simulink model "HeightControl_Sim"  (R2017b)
settings: Solver=ode4  StartTime=0.0  StopTime=2  FixedStep=0.001  RelTol=1e-3
InitFcn:
  | Init_control;
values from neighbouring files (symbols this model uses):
  DEG2RAD = 0.0174533    [Init_control.m]
  Kd_PITCH_AngleRate = 0.001    [Init_control.m]
  Kd_ROLL_AngleRate = 0.001    [Init_control.m]
  Kd_YAW_AngleRate = 0.00    (= 0)    [Init_control.m]
  Ki_PITCH_AngleRate = 0.02    [Init_control.m]
  Ki_ROLL_AngleRate = 0.02    [Init_control.m]
  Ki_YAW_AngleRate = 0.001    [Init_control.m]
  Kp_PITCH_ANGLE = 6.5    [Init_control.m]
  Kp_PITCH_AngleRate = 0.1    [Init_control.m]
  Kp_ROLL_ANGLE = 6.5    [Init_control.m]
  Kp_ROLL_AngleRate = 0.1    [Init_control.m]
  Kp_YAW_AngleRate = 0.3    [Init_control.m]
  Kpxp = 1.0    (= 1)    [Init_control.m]
  Kpyp = 1.0    (= 1)    [Init_control.m]
  Kpzp = 4.0    (= 4)    [Init_control.m]
  Kvxd = 0.01    [Init_control.m]
  Kvxi = 0.4    [Init_control.m]
  Kvxp = 2.5    [Init_control.m]
  Kvyd = 0.01    [Init_control.m]
  Kvyi = 0.4    [Init_control.m]
  Kvyp = 2.5    [Init_control.m]
  Kvzd = 0.005    [Init_control.m]
  Kvzi = 0.01    [Init_control.m]
  Kvzp = 0.45    [Init_control.m]
  MAX_CONTROL_ANGLE_PITCH = 35    [Init_control.m]
  MAX_CONTROL_ANGLE_RATE_PITCH = 220    [Init_control.m]
  MAX_CONTROL_ANGLE_RATE_ROLL = 220    [Init_control.m]
  MAX_CONTROL_ANGLE_RATE_Y = 200    [Init_control.m]
  MAX_CONTROL_ANGLE_ROLL = 35    [Init_control.m]
  MAX_CONTROL_VELOCITY_XY = 5    [Init_control.m]
  MAX_CONTROL_VELOCITY_Z = 3    [Init_control.m]
  ModelInit_AngEuler = [0, 0, 0]    [Init_control.m]    (also in Init.m)
  ModelInit_PosE = [0, 0, -100]    [Init_control.m]    (also in Init.m = [0, 0, 0])
  ModelInit_Rads = 0    [Init_control.m]    (also in Init.m)
  ModelInit_RateB = [0, 0, 0]    [Init_control.m]    (also in Init.m)
  ModelInit_VelB = [0, 0, 0]    [Init_control.m]    (also in Init.m)
  ModelParam_envGravityAcc = 9.8    [Init.m]
  ModelParam_motorCr = 1148    [Init.m]
  ModelParam_motorJm = 0.0001287    [Init.m]
  ModelParam_motorT = 0.02    [Init.m]
  ModelParam_motorWb = -141.4    [Init.m]
  ModelParam_rotorCm = 1.779e-07    [Init.m]
  ModelParam_rotorCt = 1.105e-05    [Init.m]
  ModelParam_uavCCm = [0.0035 0.0039 0.0034]    [Init.m]
  ModelParam_uavCd = 0.055    [Init.m]
  ModelParam_uavJ = [ModelParam_uavJxx, 0, 0;     0, ModelParam_uavJyy, 0;     0, 0, ModelParam_uavJzz]    [Init.m]
  ModelParam_uavMass = 1.4    [Init.m]
  ModelParam_uavR = 0.225    [Init.m]
  Saturation_I_ah = 3.43    [Init_control.m]
  Saturation_I_az = 5    [Init_control.m]
  Saturation_I_RP_Max = 0.3    [Init_control.m]
  Saturation_I_RP_Min = -0.3    [Init_control.m]
  Saturation_I_Y_Max = 0.2    [Init_control.m]
  Saturation_I_Y_Min = -0.2    [Init_control.m]
  THR_HOVER = 0.609    [Init_control.m]
undefined symbols (not defined in the file or in its folder): Column, D, DiscIntNeverNeededParam, earthRadius, Receive, Send, vector
libraries: simulink x8, aerolibfltsims x3, sharedutil x2, aerolibanimutils x1
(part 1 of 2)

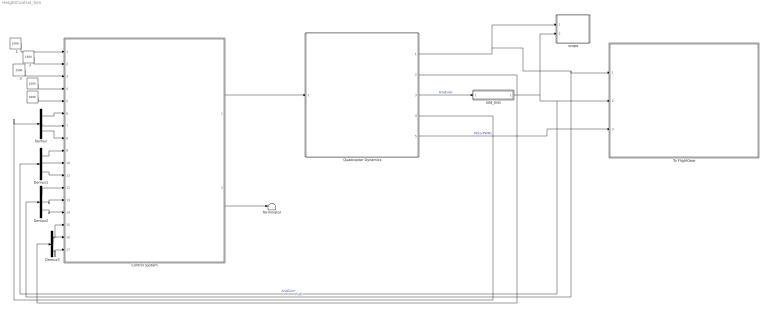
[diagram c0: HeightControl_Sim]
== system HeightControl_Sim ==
  " " : Constant  Value=1000  OutDataTypeStr=uint16
  "          " : Constant  Value=1500  OutDataTypeStr=uint16
  "   1" : Constant  Value=1500  OutDataTypeStr=uint16
  "   2" : Constant  Value=1500  OutDataTypeStr=uint16
  "   3" : Constant  Value=1500  OutDataTypeStr=uint16
  Control System : Subsystem
  Demux{,1..3} (4 alike) : Demux  Outputs=3
  Quadcopter Dynamics : Subsystem
  Terminator : Terminator
  To FlightGear : Subsystem
  add_bias : Subsystem
  scope : Subsystem
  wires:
  Quadcopter Dynamics/1(PosE) -> scope/1(Pos), To FlightGear/1(PosE), Demux2/1  "PosE"
  Quadcopter Dynamics/5(MotorRPMS) -> To FlightGear/3(MotorPWMs)  "MotorPWMs"
  Control System/2(LED) -> Terminator/1
  add_bias/1("eulerAngle ") -> scope/2(EulerAngle), To FlightGear/2(AngEuler), Demux1/1  "AngEuler"
  "          "/1 -> Control System/4(ch4)
  Quadcopter Dynamics/4(AngRateB) -> Demux/1
  " "/1 -> Control System/5(ch5)
  Demux/1 -> Control System/6(p)
  Demux/2 -> Control System/7(q)
  Demux/3 -> Control System/8(r)
  Demux2/1 -> Control System/12(x)
  Demux2/2 -> Control System/13(y)
  Demux2/3 -> Control System/14(z)
  Demux3/1 -> Control System/15(vx)
  Demux3/2 -> Control System/16(vy)
  Demux3/3 -> Control System/17(vz)
  "   1"/1 -> Control System/1(ch1)
  Quadcopter Dynamics/2(VelE) -> Demux3/1
  "   2"/1 -> Control System/2(ch2)
  Quadcopter Dynamics/3(AngEuler) -> add_bias/1(eulerAngle)  "AngEuler"
  Demux1/2 -> Control System/10(pitch)
  Demux1/1 -> Control System/9(roll)
  Demux1/3 -> Control System/11(yaw)
  "   3"/1 -> Control System/3(ch3)
  Control System/1(PWM) -> Quadcopter Dynamics/1(inPWMs)

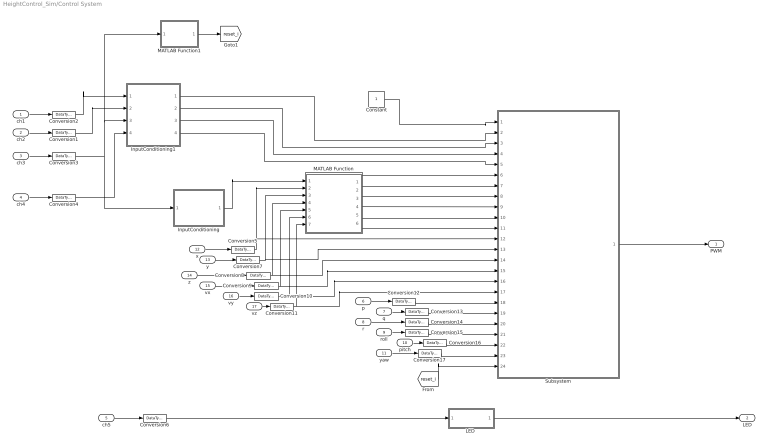
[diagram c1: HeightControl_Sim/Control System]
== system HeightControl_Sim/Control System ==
  ch1 : Inport  OutDataTypeStr=uint16  PortDimensions=1
  ch2 : Inport  Port=2  OutDataTypeStr=uint16  PortDimensions=1
  ch3 : Inport  Port=3  OutDataTypeStr=uint16  PortDimensions=1
  ch4 : Inport  Port=4  OutDataTypeStr=uint16  PortDimensions=1
  ch5 : Inport  Port=5  OutDataTypeStr=uint16  PortDimensions=1  Interpolate=off
  p : Inport  Port=6  PortDimensions=1
  q : Inport  Port=7  PortDimensions=1
  r : Inport  Port=8  PortDimensions=1
  roll : Inport  Port=9  PortDimensions=1
  pitch : Inport  Port=10  PortDimensions=1
  yaw : Inport  Port=11  PortDimensions=1
  x : Inport  Port=12
  y : Inport  Port=13
  z : Inport  Port=14
  vx : Inport  Port=15
  vy : Inport  Port=16
  vz : Inport  Port=17
  Constant : Constant
  Conversion{1..17} (17 alike) : DataTypeConversion  OutDataTypeStr=double
  InputConditioning : Subsystem
  InputConditioning1 : Subsystem
  "LED " : Subsystem
  MATLAB Function : MATLAB Function
  MATLAB Function1 : MATLAB Function  TreatAsAtomicUnit=on
  Subsystem : Subsystem
  PWM : Outport
  LED : Outport  Port=2  PortDimensions=1
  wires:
  ch3/1 -> Conversion3/1
  ch5/1 -> Conversion6/1
  ch4/1 -> Conversion4/1
  "LED "/1(Out1) -> LED/1
  Conversion6/1 -> "LED "/1(In1)
  Conversion4/1 -> InputConditioning1/4(ch4)
  ch1/1 -> Conversion2/1
  ch2/1 -> Conversion1/1
  Conversion1/1 -> InputConditioning1/2(ch2)
  x/1 -> Conversion5/1
  y/1 -> Conversion7/1
  z/1 -> Conversion8/1
  Constant/1 -> Subsystem/1(mode)
  roll/1 -> Conversion15/1
  pitch/1 -> Conversion16/1
  p/1 -> Conversion12/1
  q/1 -> Conversion13/1
  r/1 -> Conversion14/1
  yaw/1 -> Conversion17/1
  vz/1 -> Conversion11/1
  vy/1 -> Conversion10/1
  vx/1 -> Conversion9/1
  InputConditioning1/2(Roll_d) -> Subsystem/3(roll_d)
  InputConditioning1/3(Pitch_d) -> Subsystem/4(pitch_d)
  InputConditioning1/1(Thrust) -> Subsystem/2(thrust_d)
  InputConditioning1/4(yawRate_d) -> Subsystem/5(yawrate_d)
  Conversion5/1 -> Subsystem/12(x), MATLAB Function/2(x)
  Conversion7/1 -> Subsystem/13(y), MATLAB Function/3(y)
  Conversion8/1 -> Subsystem/14(z), MATLAB Function/4(z)
  Conversion9/1 -> Subsystem/15(vx), MATLAB Function/5(vx)
  Conversion10/1 -> Subsystem/16(vy), MATLAB Function/6(vy)
  Conversion11/1 -> Subsystem/17(vz), MATLAB Function/7(vz)
  Conversion12/1 -> Subsystem/18(p)
  Conversion13/1 -> Subsystem/19(q)
  Conversion14/1 -> Subsystem/20(r)
  Conversion15/1 -> Subsystem/21(roll)
  Conversion16/1 -> Subsystem/22(pitch)
  Conversion17/1 -> Subsystem/23(psi)
  Conversion3/1 -> InputConditioning1/3(ch3), MATLAB Function1/1(ch3), InputConditioning/1(z)
  MATLAB Function1/1(reset_i) -> [reset_i]
  [reset_i] -> Subsystem/24(reset_i)
  Conversion2/1 -> InputConditioning1/1("ch1 ")
  InputConditioning/1(vz) -> MATLAB Function/1(vzd)
  MATLAB Function/1(vx_d) -> Subsystem/6(vx_d)
  MATLAB Function/2(vy_d) -> Subsystem/7(vy_d)
  MATLAB Function/3(vz_d) -> Subsystem/8(vz_d)
  MATLAB Function/4(x_d) -> Subsystem/9(x_d)
  MATLAB Function/5(y_d) -> Subsystem/10(y_d)
  MATLAB Function/6(z_d) -> Subsystem/11(z_d)
  Subsystem/1(PWM) -> PWM/1

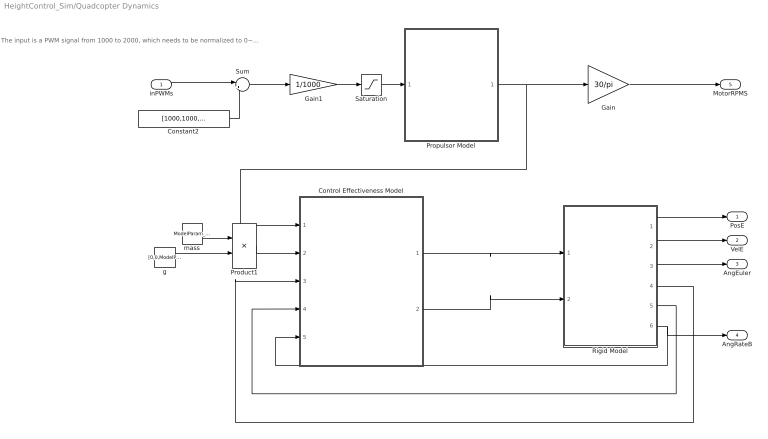
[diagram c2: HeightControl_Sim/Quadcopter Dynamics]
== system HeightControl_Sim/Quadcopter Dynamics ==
  note: The input is a PWM signal from 1000 to 2000, which needs to be normalized to 0~1.
  inPWMs : Inport
  Constant2 : Constant  Value=[1000,1000,1000,1000]
  Control Effectiveness Model : Subsystem
  Gain : Gain  Gain=30/pi
  Gain1 : Gain  Gain=1/1000
  Product1 : Product
  Propulsor Model : Subsystem
  Rigid Model : Subsystem
  Saturation : Saturate  UpperLimit=1  LowerLimit=0
  Sum : Sum  Inputs=|+-
  g : Constant  Value=[0,0,ModelParam_envGravityAcc]
  mass : Constant  Value=ModelParam_uavMass
  PosE : Outport
  VelE : Outport  Port=2
  AngEuler : Outport  Port=3
  AngRateB : Outport  Port=4
  MotorRPMS : Outport  Port=5
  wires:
  Saturation/1 -> Propulsor Model/1(inPWMs)
  Rigid Model/6("p,q,r ") -> Control Effectiveness Model/5(p.q,r), AngRateB/1
  mass/1 -> Product1/1
  Rigid Model/4(DCM) -> Control Effectiveness Model/3(DCM)
  Propulsor Model/1(MotorRads) -> Gain/1, Control Effectiveness Model/1(MotorRads)
  Gain1/1 -> Saturation/1
  Rigid Model/2(ve) -> VelE/1
  Sum/1 -> Gain1/1
  Product1/1 -> Control Effectiveness Model/2(mg)
  Rigid Model/5("vb ") -> Control Effectiveness Model/4(Vb)
  Rigid Model/1("xe ") -> PosE/1
  Rigid Model/3(Euler) -> AngEuler/1
  Control Effectiveness Model/1(Mb) -> Rigid Model/1(Mb)
  inPWMs/1 -> Sum/1
  Control Effectiveness Model/2(Fb) -> Rigid Model/2(f)
  Constant2/1 -> Sum/2
  g/1 -> Product1/2
  Gain/1 -> MotorRPMS/1

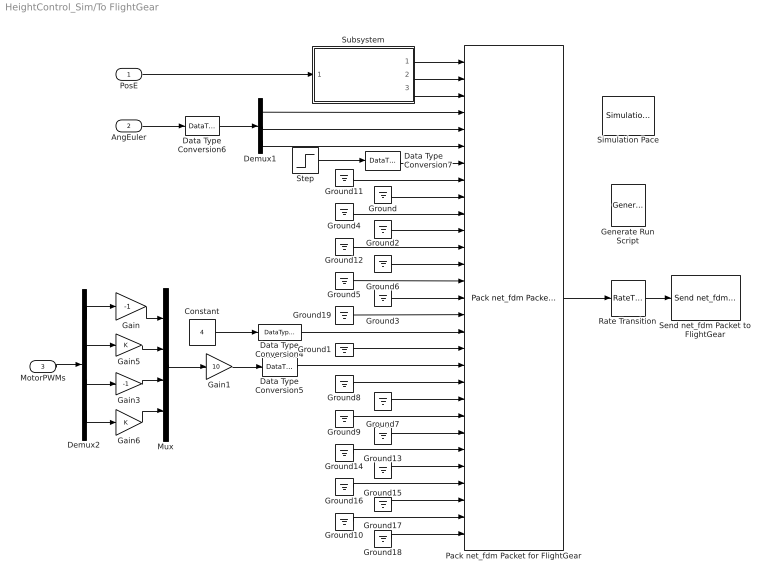
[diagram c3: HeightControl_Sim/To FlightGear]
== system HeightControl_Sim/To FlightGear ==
  PosE : Inport
  AngEuler : Inport  Port=2
  MotorPWMs : Inport  Port=3
  Constant : Constant  Value=4
  Data Type Conversion4 : DataTypeConversion  OutDataTypeStr=uint32
  Data Type Conversion5 : DataTypeConversion  OutDataTypeStr=single
  Data Type Conversion6 : DataTypeConversion  OutDataTypeStr=single
  Data Type Conversion7 : DataTypeConversion  OutDataTypeStr=single
  Demux1 : Demux  Outputs=3
  Demux2 : Demux
  Gain : Gain  Gain=-1
  Gain1 : Gain  Gain=10
  Gain3 : Gain  Gain=-1
  Gain5 : Gain
  Gain6 : Gain
  Generate Run Script : aerolibfltsims/Generate Run Script  OutputFileName=runfg_myownUAV.bat  FlightGearBaseDirectory=C:\Program Files\FlightGear 2016.1.2  GeometryModelName=myownUAV  DestinationPort=5502  OriginAddress=127.0.0.1  OriginPort=5505  LocalAddress=127.0.0.1  AirportId=KSFO  RunwayId=10L  InitialAltitude=0  InitialHeading=0  OffsetDistance=0  OffsetAzimuth=0  GenerateFile=off  Architecture=Default  dataFlow=Send-Receive
  Ground{,1..19} (20 alike) : Ground
  Mux : Mux
  Pack net_fdm Packet for FlightGear : aerolibfltsims/Pack net_fdm Packet for FlightGear  FlightGearVersion=v2016.1  ShowPositionAttitudeInputs=on  ShowVelocityAccelerationInputs=off  ShowControlSurfacePositionInputs=on  ShowEngineFuelInputs=on  ShowLandingGearInputs=off  ShowEnvironmentInputs=off  SampleTime=0.01
  Rate Transition : RateTransition
  Send net_fdm Packet to FlightGear : aerolibfltsims/Send net_fdm Packet to FlightGear  DestinationIpAddress=127.0.0.1  DestinationPort=5502  LocalIpPort=-1  varLen=off  SampleTime=0.005
  Simulation Pace : aerolibanimutils/Simulation Pace  SimulationPace=1  SleepMode=MATLAB Thread  OutputPaceError=off  SampleTime=-1
  Step : Step  Time=0  SampleTime=0
  Subsystem : Subsystem
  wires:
  Gain1/1 -> Data Type Conversion5/1
  Data Type Conversion6/1 -> Demux1/1
  Demux1/3 -> Pack net_fdm Packet for FlightGear/6
  Demux1/2 -> Pack net_fdm Packet for FlightGear/5
  Demux1/1 -> Pack net_fdm Packet for FlightGear/4
  Ground19/1 -> Pack net_fdm Packet for FlightGear/16
  Subsystem/3(h) -> Pack net_fdm Packet for FlightGear/3
  Subsystem/2(u) -> Pack net_fdm Packet for FlightGear/2
  Subsystem/1("l ") -> Pack net_fdm Packet for FlightGear/1
  PosE/1 -> Subsystem/1(In1)
  Rate Transition/1 -> Send net_fdm Packet to FlightGear/1
  Gain6/1 -> Mux/4
  Demux2/4 -> Gain6/1
  Gain5/1 -> Mux/2
  Demux2/2 -> Gain5/1
  Gain3/1 -> Mux/3
  Gain/1 -> Mux/1
  Demux2/3 -> Gain3/1
  Demux2/1 -> Gain/1
  Mux/1 -> Gain1/1
  MotorPWMs/1 -> Demux2/1
  AngEuler/1 -> Data Type Conversion6/1
  Ground12/1 -> Pack net_fdm Packet for FlightGear/12
  Ground2/1 -> Pack net_fdm Packet for FlightGear/11
  Data Type Conversion5/1 -> Pack net_fdm Packet for FlightGear/19
  Constant/1 -> Data Type Conversion4/1
  Ground11/1 -> Pack net_fdm Packet for FlightGear/8
  Ground4/1 -> Pack net_fdm Packet for FlightGear/10
  Ground6/1 -> Pack net_fdm Packet for FlightGear/13
  Ground5/1 -> Pack net_fdm Packet for FlightGear/14
  Ground3/1 -> Pack net_fdm Packet for FlightGear/15
  Ground1/1 -> Pack net_fdm Packet for FlightGear/18
  Data Type Conversion4/1 -> Pack net_fdm Packet for FlightGear/17
  Step/1 -> Data Type Conversion7/1
  Ground18/1 -> Pack net_fdm Packet for FlightGear/29
  Ground10/1 -> Pack net_fdm Packet for FlightGear/28
  Ground17/1 -> Pack net_fdm Packet for FlightGear/27
  Ground16/1 -> Pack net_fdm Packet for FlightGear/26
  Ground15/1 -> Pack net_fdm Packet for FlightGear/25
  Ground14/1 -> Pack net_fdm Packet for FlightGear/24
  Ground13/1 -> Pack net_fdm Packet for FlightGear/23
  Ground9/1 -> Pack net_fdm Packet for FlightGear/22
  Ground7/1 -> Pack net_fdm Packet for FlightGear/21
  Ground/1 -> Pack net_fdm Packet for FlightGear/9
  Ground8/1 -> Pack net_fdm Packet for FlightGear/20
  Data Type Conversion7/1 -> Pack net_fdm Packet for FlightGear/7
  Pack net_fdm Packet for FlightGear/1 -> Rate Transition/1

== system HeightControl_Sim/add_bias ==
  eulerAngle : Inport
  Constant : Constant  Value=0.03
  Constant1 : Constant  Value=0.03
  Demux4 : Demux  Outputs=3
  Mux : Mux  Inputs=3
  Sum : Sum  Inputs=|++
  Sum1 : Sum  Inputs=|++
  "eulerAngle " : Outport
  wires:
  Sum/1 -> Mux/1
  eulerAngle/1 -> Demux4/1
  Sum1/1 -> Mux/2
  Demux4/3 -> Mux/3  "yaw"
  Demux4/2 -> Sum1/1  "pitch"
  Constant/1 -> Sum/2
  Demux4/1 -> Sum/1  "roll"
  Constant1/1 -> Sum1/2
  Mux/1 -> "eulerAngle "/1

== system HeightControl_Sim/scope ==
  Pos : Inport
  EulerAngle : Inport  Port=2
  Demux1 : Demux  Outputs=3
  Demux4 : Demux  Outputs=3
  Terminator : Terminator
  XY : simulink/Sinks/XY Graph  xmin=-0.5  xmax=1  ymin=-1  ymax=0.5  st=-1
  rp : Scope  NumInputPorts=2
  z : Scope
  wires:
  Demux1/1 -> XY/1
  Demux4/2 -> rp/2
  Demux4/1 -> rp/1
  Demux4/3 -> Terminator/1
  EulerAngle/1 -> Demux4/1
  Pos/1 -> Demux1/1
  Demux1/3 -> z/1
  Demux1/2 -> XY/2

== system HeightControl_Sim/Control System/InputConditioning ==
  z : Inport
  Saturation10 : Saturate  UpperLimit=1  LowerLimit=-1
  deadzone1 : MATLAB Function  TreatAsAtomicUnit=on
  max_vz : Gain  Gain=-MAX_CONTROL_VELOCITY_Z  OutDataTypeStr=Inherit: Inherit via back propagation
  vz : Outport
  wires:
  Saturation10/1 -> max_vz/1
  deadzone1/1(y) -> Saturation10/1
  max_vz/1 -> vz/1
  z/1 -> deadzone1/1(u)

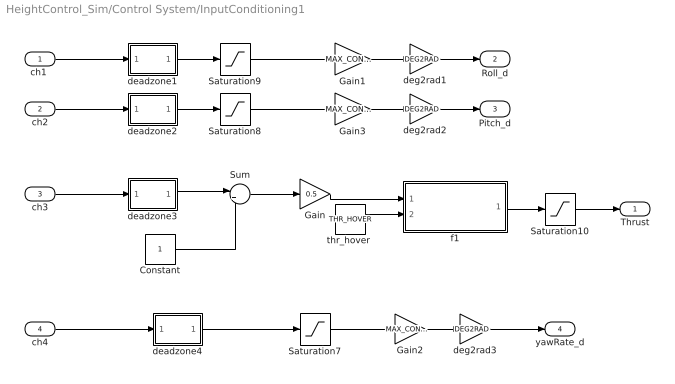
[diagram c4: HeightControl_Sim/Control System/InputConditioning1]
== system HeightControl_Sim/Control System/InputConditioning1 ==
  "ch1 " : Inport
  ch2 : Inport  Port=2
  ch3 : Inport  Port=3
  ch4 : Inport  Port=4
  Constant : Constant
  Gain : Gain  Gain=0.5
  Gain1 : Gain  Gain=MAX_CONTROL_ANGLE_ROLL  OutDataTypeStr=Inherit: Inherit via back propagation
  Gain2 : Gain  Gain=MAX_CONTROL_ANGLE_RATE_Y
  Gain3 : Gain  Gain=MAX_CONTROL_ANGLE_PITCH  OutDataTypeStr=Inherit: Inherit via back propagation
  Saturation10 : Saturate  UpperLimit=1  LowerLimit=0
  Saturation7 : Saturate  UpperLimit=1  LowerLimit=-1
  Saturation8 : Saturate  UpperLimit=1  LowerLimit=-1
  Saturation9 : Saturate  UpperLimit=1  LowerLimit=-1
  Sum : Sum  Inputs=|++
  deadzone1 : MATLAB Function  TreatAsAtomicUnit=on
  deadzone2 : MATLAB Function  TreatAsAtomicUnit=on
  deadzone3 : MATLAB Function  TreatAsAtomicUnit=on
  deadzone4 : MATLAB Function  TreatAsAtomicUnit=on
  deg2rad1 : Gain  Gain=DEG2RAD
  deg2rad2 : Gain  Gain=DEG2RAD
  deg2rad3 : Gain  Gain=DEG2RAD
  f1 : MATLAB Function  TreatAsAtomicUnit=on
  "thr_hover " : Constant  Value=THR_HOVER
  Thrust : Outport
  Roll_d : Outport  Port=2
  Pitch_d : Outport  Port=3
  yawRate_d : Outport  Port=4
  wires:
  deadzone3/1(y) -> Sum/1
  ch3/1 -> deadzone3/1(u)
  deadzone2/1(y) -> Saturation8/1
  Saturation10/1 -> Thrust/1
  deadzone1/1(y) -> Saturation9/1
  "ch1 "/1 -> deadzone1/1(u)
  ch2/1 -> deadzone2/1(u)
  Saturation9/1 -> Gain1/1
  Saturation8/1 -> Gain3/1
  Gain3/1 -> deg2rad2/1
  Constant/1 -> Sum/2
  Sum/1 -> Gain/1
  Gain1/1 -> deg2rad1/1
  deg2rad1/1 -> Roll_d/1
  deg2rad2/1 -> Pitch_d/1
  Saturation7/1 -> Gain2/1
  deadzone4/1(y) -> Saturation7/1
  ch4/1 -> deadzone4/1(u)
  Gain2/1 -> deg2rad3/1
  deg2rad3/1 -> yawRate_d/1
  "thr_hover "/1 -> f1/2(hover)
  Gain/1 -> f1/1(in)
  f1/1(y) -> Saturation10/1

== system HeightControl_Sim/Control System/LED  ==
  In1 : Inport
  Compare To Constant3 : simulink/Logic and Bit Operations/Compare To Constant  relop=>=  const=uint16(1500)  OutDataTypeStr=boolean
  Out1 : Outport
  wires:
  Compare To Constant3/1 -> Out1/1
  In1/1 -> Compare To Constant3/1

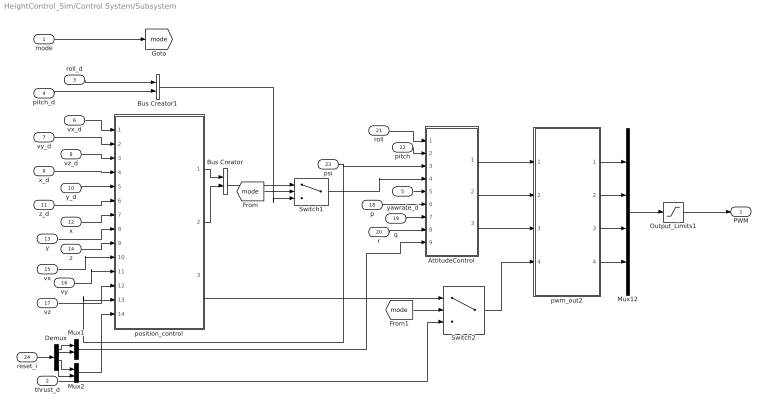
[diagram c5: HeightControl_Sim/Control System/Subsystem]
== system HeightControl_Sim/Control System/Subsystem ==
  mode : Inport
  thrust_d : Inport  Port=2
  roll_d : Inport  Port=3
  pitch_d : Inport  Port=4
  yawrate_d : Inport  Port=5
  vx_d : Inport  Port=6
  vy_d : Inport  Port=7
  vz_d : Inport  Port=8
  x_d : Inport  Port=9
  y_d : Inport  Port=10
  z_d : Inport  Port=11
  x : Inport  Port=12
  y : Inport  Port=13
  z : Inport  Port=14
  vx : Inport  Port=15
  vy : Inport  Port=16
  vz : Inport  Port=17
  p : Inport  Port=18  PortDimensions=1
  q : Inport  Port=19  PortDimensions=1
  r : Inport  Port=20  PortDimensions=1
  roll : Inport  Port=21  PortDimensions=1
  pitch : Inport  Port=22  PortDimensions=1
  psi : Inport  Port=23  PortDimensions=1
  reset_i : Inport  Port=24
  AttitudeControl : Subsystem
  Bus Creator : BusCreator  Inputs=2
  Bus Creator1 : BusCreator  Inputs=2
  Demux : Demux
  Mux1 : Mux  Inputs=2
  Mux12 : Mux
  Mux2 : Mux  Inputs=2
  Output_Limits1 : Saturate  UpperLimit=2000  LowerLimit=1000
  Switch1 : Switch  Threshold=2
  Switch2 : Switch  Threshold=1
  position_control : Subsystem
  pwm_out2 : MATLAB Function  SystemSampleTime=0.004
  PWM : Outport
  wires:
  pwm_out2/4(M4) -> Mux12/4
  pwm_out2/3(M3) -> Mux12/3
  yawrate_d/1 -> AttitudeControl/5(yaw)
  roll/1 -> AttitudeControl/1(phi)
  Output_Limits1/1 -> PWM/1
  q/1 -> AttitudeControl/7(q)
  AttitudeControl/1(Roll) -> pwm_out2/1(Roll)
  pwm_out2/2(M2) -> Mux12/2
  AttitudeControl/2(Pitch) -> pwm_out2/2(Pitch)
  pitch/1 -> AttitudeControl/2(theta)
  Mux12/1 -> Output_Limits1/1
  position_control/2(theta) -> Bus Creator/2
  pwm_out2/1(M1) -> Mux12/1
  AttitudeControl/3(Yaw) -> pwm_out2/3(Yaw)
  position_control/1(phi) -> Bus Creator/1
  p/1 -> AttitudeControl/6(p)
  vx/1 -> position_control/10(vx)
  vz/1 -> position_control/12(vz)
  vy/1 -> position_control/11(vy)
  x_d/1 -> position_control/4(x_desired)
  y_d/1 -> position_control/5(y_desired)
  z_d/1 -> position_control/6(z_desired)
  mode/1 -> [mode]
  vz_d/1 -> position_control/3(vz_desired)
  x/1 -> position_control/7(x)
  vx_d/1 -> position_control/1(vx_desired)
  vy_d/1 -> position_control/2(vy_desired)
  y/1 -> position_control/8(y)
  z/1 -> position_control/9(z)
  Bus Creator/1 -> Switch1/1
  [mode] -> Switch1/2
  Switch1/1 -> AttitudeControl/4(roll_pitch)
  roll_d/1 -> Bus Creator1/1
  pitch_d/1 -> Bus Creator1/2
  Bus Creator1/1 -> Switch1/3
  [mode] -> Switch2/2
  position_control/3(thr) -> Switch2/1
  Switch2/1 -> pwm_out2/4(Thrust)
  thrust_d/1 -> Switch2/3
  r/1 -> AttitudeControl/8(r)
  psi/1 -> AttitudeControl/3(psi), position_control/13(psi)
  reset_i/1 -> Demux/1
  Mux2/1 -> position_control/14(reset_i)
  Mux1/1 -> AttitudeControl/9(reset_i)
  Demux/1 -> Mux1/1
  Demux/2 -> Mux1/2
  Demux/3 -> Mux2/1
  Demux/4 -> Mux2/2

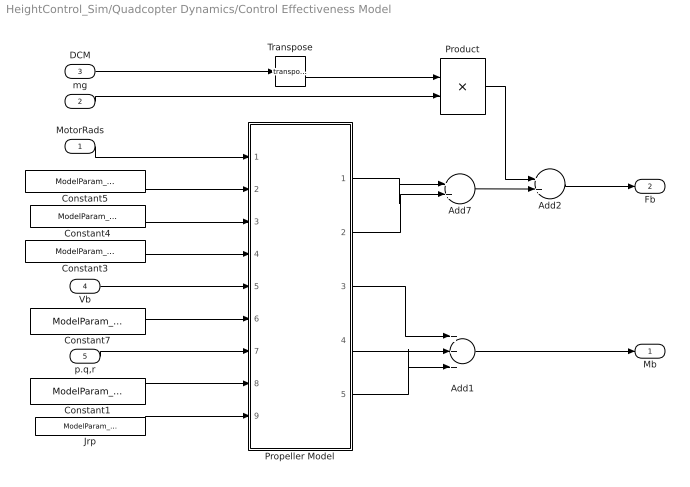
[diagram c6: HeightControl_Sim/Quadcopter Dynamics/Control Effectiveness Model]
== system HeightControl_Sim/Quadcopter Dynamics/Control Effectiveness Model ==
  MotorRads : Inport
  mg : Inport  Port=2
  DCM : Inport  Port=3
  Vb : Inport  Port=4
  p.q,r : Inport  Port=5
  Add1 : Sum  Inputs=+++
  Add2 : Sum
  Add7 : Sum
  Constant1 : Constant  Value=ModelParam_uavCCm
  Constant3 : Constant  Value=ModelParam_rotorCt
  Constant4 : Constant  Value=ModelParam_rotorCm
  Constant5 : Constant  Value=ModelParam_uavR
  Constant7 : Constant  Value=ModelParam_uavCd
  Jrp : Constant  Value=ModelParam_motorJm
  Product : Product  Multiplication=Matrix(*)
  Propeller Model : MATLAB Function  TreatAsAtomicUnit=on
  Transpose : Math  Operator=transpose
  Mb : Outport
  Fb : Outport  Port=2
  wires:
  Add2/1 -> Fb/1
  Constant3/1 -> Propeller Model/4(Ct)
  Propeller Model/2(Fd) -> Add7/2
  Add7/1 -> Add2/2
  Propeller Model/1(Fb) -> Add7/1
  Product/1 -> Add2/1
  mg/1 -> Product/2
  DCM/1 -> Transpose/1
  Constant7/1 -> Propeller Model/6(Cd)
  Vb/1 -> Propeller Model/5(Vb)
  Constant5/1 -> Propeller Model/2(R)
  Constant4/1 -> Propeller Model/3(Cm)
  MotorRads/1 -> Propeller Model/1(w)
  Transpose/1 -> Product/1
  Propeller Model/3(Mb) -> Add1/1
  Propeller Model/4(Md) -> Add1/2
  Add1/1 -> Mb/1
  p.q,r/1 -> Propeller Model/7(wb)
  Constant1/1 -> Propeller Model/8(Cdm)
  Jrp/1 -> Propeller Model/9(Jrp)
  Propeller Model/5(Ga) -> Add1/3

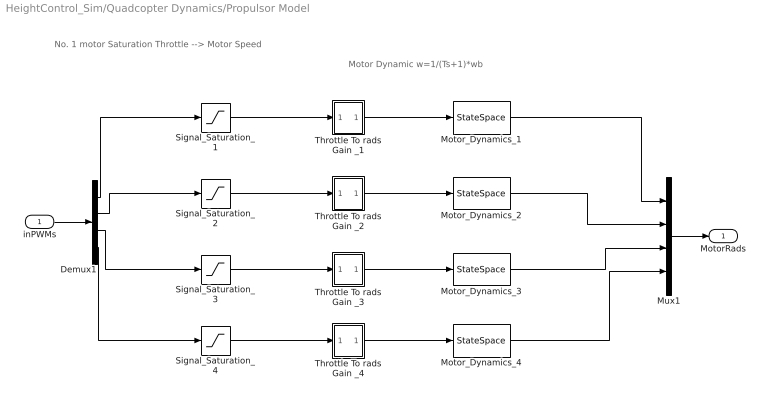
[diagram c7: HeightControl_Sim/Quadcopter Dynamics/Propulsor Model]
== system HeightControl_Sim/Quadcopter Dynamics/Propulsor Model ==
  note: Motor Dynamic w=1/(Ts+1)*wb
  note: No. 1 motor Saturation Throttle --> Motor Speed
  inPWMs : Inport
  Demux1 : Demux
  Motor_Dynamics_{1..4} (4 alike) : StateSpace  A=-1/ModelParam_motorT  C=1/ModelParam_motorT  D=0  InitialCondition=ModelInit_Rads*ModelParam_motorT
  Mux1 : Mux
  Signal_Saturation_{1..4} (4 alike) : Saturate  UpperLimit=1  LowerLimit=0
  Throttle To rads Gain _1 : Subsystem
  Throttle To rads Gain _2 : Subsystem
  Throttle To rads Gain _3 : Subsystem
  Throttle To rads Gain _4 : Subsystem
  MotorRads : Outport
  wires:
  Throttle To rads Gain _4/1(Out5) -> Motor_Dynamics_4/1
  Signal_Saturation_4/1 -> Throttle To rads Gain _4/1(In5)
  Signal_Saturation_3/1 -> Throttle To rads Gain _3/1(In5)
  Signal_Saturation_2/1 -> Throttle To rads Gain _2/1(In5)
  Motor_Dynamics_4/1 -> Mux1/4
  Motor_Dynamics_3/1 -> Mux1/3
  Motor_Dynamics_2/1 -> Mux1/2
  Motor_Dynamics_1/1 -> Mux1/1
  Signal_Saturation_1/1 -> Throttle To rads Gain _1/1(In5)
  Mux1/1 -> MotorRads/1
  Throttle To rads Gain _3/1(Out5) -> Motor_Dynamics_3/1
  Throttle To rads Gain _2/1(Out5) -> Motor_Dynamics_2/1
  Throttle To rads Gain _1/1(Out5) -> Motor_Dynamics_1/1
  inPWMs/1 -> Demux1/1
  Demux1/4 -> Signal_Saturation_4/1
  Demux1/3 -> Signal_Saturation_3/1
  Demux1/2 -> Signal_Saturation_2/1
  Demux1/1 -> Signal_Saturation_1/1

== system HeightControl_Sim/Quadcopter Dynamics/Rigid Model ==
  Mb : Inport
  f : Inport  Port=2
  Rigid-Body Dynamic Model : Subsystem
  "Rigid-Body Kinematic Model " : Subsystem
  "xe " : Outport
  ve : Outport  Port=2
  Euler : Outport  Port=3
  DCM : Outport  Port=4
  "vb " : Outport  Port=5
  "p,q,r " : Outport  Port=6
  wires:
  Rigid-Body Dynamic Model/1("p,q,r ") -> "Rigid-Body Kinematic Model "/1(pqr), "p,q,r "/1
  "Rigid-Body Kinematic Model "/1(Euler) -> Euler/1
  "Rigid-Body Kinematic Model "/3(DCM) -> Rigid-Body Dynamic Model/3(DCM), DCM/1
  Mb/1 -> Rigid-Body Dynamic Model/1(Mb)
  f/1 -> Rigid-Body Dynamic Model/2(f)
  Rigid-Body Dynamic Model/2(ve) -> "Rigid-Body Kinematic Model "/2(ve), ve/1
  Rigid-Body Dynamic Model/3("vb ") -> "vb "/1
  "Rigid-Body Kinematic Model "/2("xe ") -> "xe "/1

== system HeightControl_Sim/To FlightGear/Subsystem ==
  In1 : Inport
  Constant1 : Constant  Value=5  VectorParams1D=off
  Constant2 : Constant  Value=-2.1361  VectorParams1D=off
  Constant3 : Constant  Value=0.65673  VectorParams1D=off
  Demux : Demux  Outputs=3
  Gain1 : Gain  Gain=10/earthRadius
  Gain2 : Gain  Gain=10/earthRadius
  Gain4 : Gain
  Gain8 : Gain  Gain=-10
  Sum10 : Sum  Inputs=|++
  Sum8 : Sum  Inputs=|++
  Sum9 : Sum  Inputs=|++
  "l " : Outport
  u : Outport  Port=2
  h : Outport  Port=3
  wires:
  Sum8/1 -> "l "/1
  In1/1 -> Demux/1
  Sum9/1 -> u/1
  Sum10/1 -> h/1
  Gain4/1 -> Gain2/1
  Demux/2 -> Gain1/1
  Gain8/1 -> Sum10/1
  Gain1/1 -> Sum8/1
  Gain2/1 -> Sum9/1
  Constant2/1 -> Sum8/2
  Demux/3 -> Gain8/1
  Demux/1 -> Gain4/1
  Constant1/1 -> Sum10/2
  Constant3/1 -> Sum9/2

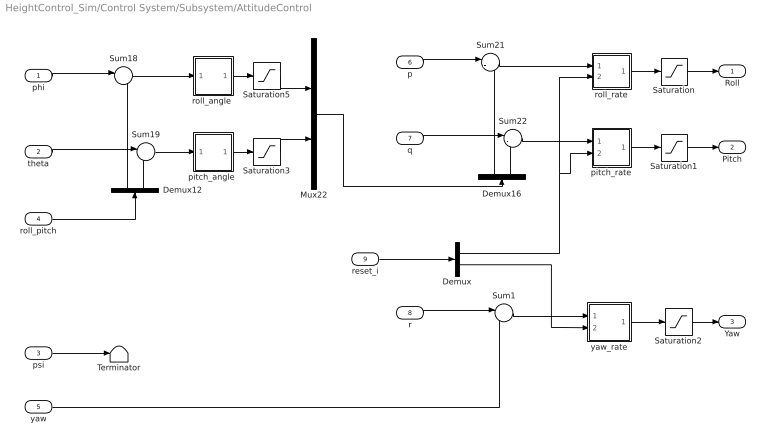
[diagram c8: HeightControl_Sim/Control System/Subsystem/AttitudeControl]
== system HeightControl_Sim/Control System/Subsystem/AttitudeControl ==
  phi : Inport
  theta : Inport  Port=2
  psi : Inport  Port=3
  roll_pitch : Inport  Port=4
  yaw : Inport  Port=5
  p : Inport  Port=6
  q : Inport  Port=7
  r : Inport  Port=8
  reset_i : Inport  Port=9
  Demux : Demux  Outputs=2
  Demux12 : Demux  Outputs=2
  Demux16 : Demux  Outputs=2
  Mux22 : Mux  Inputs=2
  Saturation : Saturate  UpperLimit=1  LowerLimit=-1
  Saturation1 : Saturate  UpperLimit=1  LowerLimit=-1
  Saturation2 : Saturate
  Saturation3 : Saturate  UpperLimit=MAX_CONTROL_ANGLE_RATE_PITCH  LowerLimit=-MAX_CONTROL_ANGLE_RATE_PITCH
  Saturation5 : Saturate  UpperLimit=MAX_CONTROL_ANGLE_RATE_ROLL  LowerLimit=-MAX_CONTROL_ANGLE_RATE_ROLL
  Sum1 : Sum  Inputs=|-+
  Sum18 : Sum  Inputs=|-+  OutMin=-90  OutMax=90
  Sum19 : Sum  Inputs=|-+  OutMin=-90  OutMax=90
  Sum21 : Sum  Inputs=|-+
  Sum22 : Sum  Inputs=|-+
  Terminator : Terminator
  "pitch_angle " : Subsystem
  pitch_rate : Subsystem
  "roll_angle " : Subsystem
  roll_rate : Subsystem
  yaw_rate : Subsystem
  Roll : Outport
  Pitch : Outport  Port=2
  Yaw : Outport  Port=3
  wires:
  Sum19/1 -> "pitch_angle "/1(x)
  "pitch_angle "/1(y) -> Saturation3/1
  Demux12/1 -> Sum18/2
  Demux12/2 -> Sum19/2
  phi/1 -> Sum18/1
  theta/1 -> Sum19/1
  Sum18/1 -> "roll_angle "/1(x)
  Sum22/1 -> pitch_rate/1(x)
  p/1 -> Sum21/1
  q/1 -> Sum22/1
  Sum21/1 -> roll_rate/1(x)
  Demux16/1 -> Sum21/2
  pitch_rate/1(y) -> Saturation1/1
  roll_rate/1(y) -> Saturation/1
  yaw_rate/1(y) -> Saturation2/1
  roll_pitch/1 -> Demux12/1
  Saturation/1 -> Roll/1
  Saturation1/1 -> Pitch/1
  Saturation2/1 -> Yaw/1
  Demux16/2 -> Sum22/2
  Mux22/1 -> Demux16/1
  r/1 -> Sum1/1
  Sum1/1 -> yaw_rate/1(x)
  "roll_angle "/1(y) -> Saturation5/1
  Saturation5/1 -> Mux22/1
  Saturation3/1 -> Mux22/2
  yaw/1 -> Sum1/2
  Demux/1 -> roll_rate/2(reset_i), pitch_rate/2(reset_i)
  reset_i/1 -> Demux/1
  Demux/2 -> yaw_rate/2(reset_i)
  psi/1 -> Terminator/1

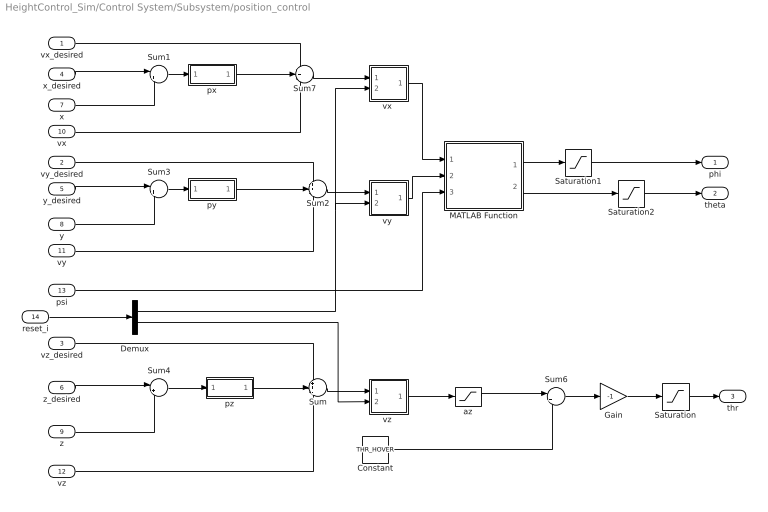
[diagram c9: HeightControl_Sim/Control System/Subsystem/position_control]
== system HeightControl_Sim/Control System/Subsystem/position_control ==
  vx_desired : Inport
  vy_desired : Inport  Port=2
  vz_desired : Inport  Port=3
  x_desired : Inport  Port=4
  y_desired : Inport  Port=5
  z_desired : Inport  Port=6
  x : Inport  Port=7
  y : Inport  Port=8
  z : Inport  Port=9
  vx : Inport  Port=10
  vy : Inport  Port=11
  vz : Inport  Port=12
  psi : Inport  Port=13
  reset_i : Inport  Port=14
  Constant : Constant  Value=THR_HOVER
  Demux : Demux  Outputs=2
  Gain : Gain  Gain=-1
  MATLAB Function : MATLAB Function  TreatAsAtomicUnit=on
  Saturation : Saturate  UpperLimit=0.9  LowerLimit=0
  Saturation1 : Saturate  UpperLimit=MAX_CONTROL_ANGLE_ROLL*DEG2RAD  LowerLimit=-MAX_CONTROL_ANGLE_ROLL*DEG2RAD
  Saturation2 : Saturate  UpperLimit=MAX_CONTROL_ANGLE_PITCH*DEG2RAD/2  LowerLimit=-MAX_CONTROL_ANGLE_PITCH*DEG2RAD/2
  Sum : Sum  Inputs=++-
  Sum{1,3..4,6} (4 alike) : Sum  Inputs=|+-
  Sum2 : Sum  Inputs=++-
  Sum7 : Sum  Inputs=++-
  az : Saturate  UpperLimit=0.4  LowerLimit=-0.4
  px : Subsystem
  py : Subsystem
  pz : Subsystem
  "vx " : Subsystem
  "vy " : Subsystem
  "vz " : Subsystem
  phi : Outport
  theta : Outport  Port=2
  thr : Outport  Port=3
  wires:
  Saturation/1 -> thr/1
  Gain/1 -> Saturation/1
  Sum6/1 -> Gain/1
  "vz "/1(y) -> az/1
  Sum4/1 -> pz/1(ez)
  z/1 -> Sum4/2
  Constant/1 -> Sum6/2
  Sum/1 -> "vz "/1(x)
  vz/1 -> Sum/3
  vx/1 -> Sum7/3
  x/1 -> Sum1/2
  y/1 -> Sum3/2
  Sum3/1 -> py/1(ey)
  y_desired/1 -> Sum3/1
  vy/1 -> Sum2/3
  Sum2/1 -> "vy "/1(x)
  Sum7/1 -> "vx "/1(x)
  Sum1/1 -> px/1(ex)
  vy_desired/1 -> Sum2/1
  py/1(vyd) -> Sum2/2
  pz/1(vzd) -> Sum/2
  z_desired/1 -> Sum4/1
  vz_desired/1 -> Sum/1
  "vx "/1(y) -> MATLAB Function/1(eax)
  px/1(vxd) -> Sum7/2
  Saturation1/1 -> phi/1
  Saturation2/1 -> theta/1
  x_desired/1 -> Sum1/1
  vx_desired/1 -> Sum7/1
  "vy "/1(y) -> MATLAB Function/2(eay)
  psi/1 -> MATLAB Function/3(psi)
  MATLAB Function/1(phi) -> Saturation1/1
  MATLAB Function/2(theta) -> Saturation2/1
  reset_i/1 -> Demux/1
  Demux/1 -> "vy "/2(reset_i), "vx "/2(reset_i)
  Demux/2 -> "vz "/2(reset_i)
  az/1 -> Sum6/1

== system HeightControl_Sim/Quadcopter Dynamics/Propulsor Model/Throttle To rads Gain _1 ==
  In5 : Inport
  Constant : Constant  Value=ModelParam_motorWb
  Gain : Gain  Gain=ModelParam_motorCr
  Sum1 : Sum  Inputs=++|
  Out5 : Outport
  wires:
  Constant/1 -> Sum1/1
  Gain/1 -> Sum1/2
  In5/1 -> Gain/1
  Sum1/1 -> Out5/1

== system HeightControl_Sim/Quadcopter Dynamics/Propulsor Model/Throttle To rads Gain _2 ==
  In5 : Inport
  Constant : Constant  Value=ModelParam_motorWb
  Gain : Gain  Gain=ModelParam_motorCr
  Sum1 : Sum  Inputs=++|
  Out5 : Outport
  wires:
  Sum1/1 -> Out5/1
  In5/1 -> Gain/1
  Gain/1 -> Sum1/2
  Constant/1 -> Sum1/1

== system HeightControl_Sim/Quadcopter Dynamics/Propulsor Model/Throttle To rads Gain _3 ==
  In5 : Inport
  Constant : Constant  Value=ModelParam_motorWb
  Gain : Gain  Gain=ModelParam_motorCr
  Sum1 : Sum  Inputs=++|
  Out5 : Outport
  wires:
  Constant/1 -> Sum1/1
  Gain/1 -> Sum1/2
  In5/1 -> Gain/1
  Sum1/1 -> Out5/1

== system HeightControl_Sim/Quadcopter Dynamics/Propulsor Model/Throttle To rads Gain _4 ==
  In5 : Inport
  Constant : Constant  Value=ModelParam_motorWb
  Gain : Gain  Gain=ModelParam_motorCr
  Sum1 : Sum  Inputs=++|
  Out5 : Outport
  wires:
  Sum1/1 -> Out5/1
  In5/1 -> Gain/1
  Gain/1 -> Sum1/2
  Constant/1 -> Sum1/1

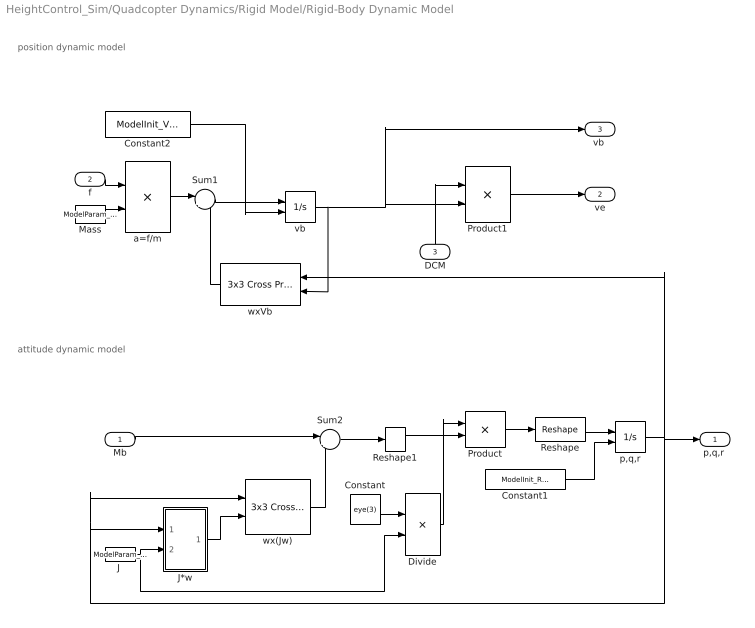
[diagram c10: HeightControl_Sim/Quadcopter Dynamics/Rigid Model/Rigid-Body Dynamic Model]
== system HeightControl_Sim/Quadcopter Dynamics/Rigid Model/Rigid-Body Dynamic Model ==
  note: attitude dynamic model
  note: position dynamic model
  Mb : Inport
  f : Inport  Port=2
  DCM : Inport  Port=3
  " Mass " : Constant  Value=ModelParam_uavMass
  Constant : Constant  Value=eye(3)
  Constant1 : Constant  Value=ModelInit_RateB
  Constant2 : Constant  Value=ModelInit_VelB
  Divide : Product  Inputs=*/  Multiplication=Matrix(*)
  "J " : Constant  Value=ModelParam_uavJ
  J*w : Subsystem
  Product : Product  Multiplication=Matrix(*)
  Product1 : Product  Multiplication=Matrix(*)
  Reshape : Reshape  OutputDimensionality=Customize  OutputDimensions=[3,1]
  Reshape1 : Reshape  OutputDimensionality=Column vector (2-D)
  Sum1 : Sum  Inputs=|+-
  Sum2 : Sum  Inputs=|+-
  a=f/m : Product  Inputs=*/
  p,q,r : Integrator  InitialConditionSource=external
  vb : Integrator  InitialConditionSource=external
  wx(Jw) : sharedutil/3x3 Cross Product
  wxVb : sharedutil/3x3 Cross Product
  "p,q,r " : Outport
  ve : Outport  Port=2
  "vb " : Outport  Port=3
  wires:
  Product/1 -> Reshape/1
  Reshape1/1 -> Product/2
  Constant/1 -> Divide/1
  Divide/1 -> Product/1
  Sum2/1 -> Reshape1/1
  "J "/1 -> Divide/2, J*w/2(J)
  p,q,r/1 -> "p,q,r "/1, J*w/1(p q r), wx(Jw)/1, wxVb/1
  J*w/1("J*w ") -> wx(Jw)/2
  Mb/1 -> Sum2/1
  wx(Jw)/1 -> Sum2/2
  Constant2/1 -> vb/2
  f/1 -> a=f/m/1
  Product1/1 -> ve/1
  wxVb/1 -> Sum1/2
  a=f/m/1 -> Sum1/1
  Sum1/1 -> vb/1
  vb/1 -> Product1/2, "vb "/1, wxVb/2
  " Mass "/1 -> a=f/m/2
  DCM/1 -> Product1/1
  Reshape/1 -> p,q,r/1
  Constant1/1 -> p,q,r/2

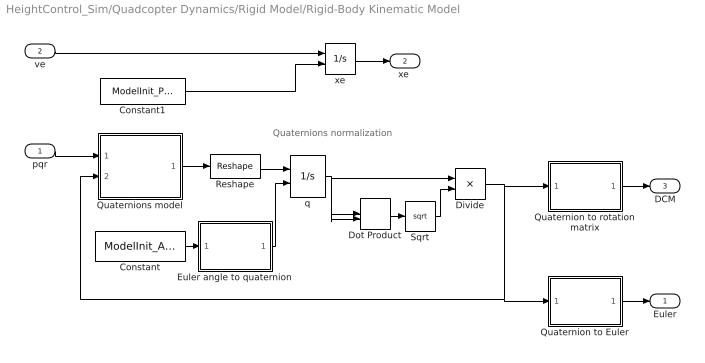
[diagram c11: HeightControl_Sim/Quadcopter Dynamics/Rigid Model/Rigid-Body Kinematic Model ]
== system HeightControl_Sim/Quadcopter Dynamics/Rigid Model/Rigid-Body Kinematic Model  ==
  note: Quaternions normalization
  pqr : Inport
  ve : Inport  Port=2
  Constant : Constant  Value=ModelInit_AngEuler
  Constant1 : Constant  Value=ModelInit_PosE
  Divide : Product  Inputs=*/
  Dot Product : DotProduct
  Euler angle to quaternion : MATLAB Function
  Quaternion to Euler : MATLAB Function
  Quaternion to rotation matrix : MATLAB Function
  Quaternions model : MATLAB Function  TreatAsAtomicUnit=on
  Reshape : Reshape  OutputDimensionality=Customize  OutputDimensions=[4,1]
  Sqrt : Sqrt
  q : Integrator  InitialConditionSource=external
  xe : Integrator  InitialConditionSource=external
  Euler : Outport
  "xe " : Outport  Port=2
  DCM : Outport  Port=3
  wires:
  Divide/1 -> Quaternion to rotation matrix/1(q), Quaternions model/2(q), Quaternion to Euler/1(q)
  Dot Product/1 -> Sqrt/1
  pqr/1 -> Quaternions model/1(pqr)
  q/1 -> Divide/1, Dot Product/1, Dot Product/2
  Quaternions model/1(qdot) -> Reshape/1
  Quaternion to rotation matrix/1(Reb) -> DCM/1
  Quaternion to Euler/1(y) -> Euler/1
  Constant/1 -> Euler angle to quaternion/1(EulerAngle)
  Euler angle to quaternion/1(q) -> q/2
  Reshape/1 -> q/1
  ve/1 -> xe/1
  xe/1 -> "xe "/1
  Constant1/1 -> xe/2
  Sqrt/1 -> Divide/2

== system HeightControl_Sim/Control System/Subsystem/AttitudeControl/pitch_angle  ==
  x : Inport
  Gain : Gain  Gain=Kp_PITCH_ANGLE
  y : Outport  InitialOutput=0
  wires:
  x/1 -> Gain/1
  Gain/1 -> y/1

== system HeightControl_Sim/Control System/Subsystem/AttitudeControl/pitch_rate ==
  x : Inport
  reset_i : Inport  Port=2
  Derivative Gain : Gain  DisableCoverage=on  Gain=Kd_PITCH_AngleRate  ParamMin=-100  ParamMax=100  OutMin=-100  OutMax=100
  Discrete Derivative : simulink/Discrete/Discrete Derivative  gainval=1.0  ICPrevScaledInput=0.0  OutMin=[]  OutMax=[]  OutDataType=fixdt(1, 16)  OutScaling=2^-10  DoSatur=off
  Discrete-Time Integrator : DiscreteIntegrator  ExternalReset=level  InitialConditionSetting=State (most efficient)  SampleTime=-1  LimitOutput=on  UpperSaturationLimit=Saturation_I_RP_Max  LowerSaturationLimit=Saturation_I_RP_Min  ICPrevOutput=DiscIntNeverNeededParam  ICPrevScaledInput=DiscIntNeverNeededParam
  Gain : Gain  Gain=Kp_PITCH_AngleRate
  Integral Gain : Gain  DisableCoverage=on  Gain=Ki_PITCH_AngleRate
  Sum : Sum  Inputs=+++
  y : Outport  InitialOutput=0
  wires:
  Discrete-Time Integrator/1 -> Sum/2
  Discrete Derivative/1 -> Sum/3
  Sum/1 -> y/1
  Gain/1 -> Sum/1
  Derivative Gain/1 -> Discrete Derivative/1
  Integral Gain/1 -> Discrete-Time Integrator/1
  x/1 -> Derivative Gain/1, Integral Gain/1, Gain/1
  reset_i/1 -> Discrete-Time Integrator/2

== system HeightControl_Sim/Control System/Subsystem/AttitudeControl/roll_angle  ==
  x : Inport
  Gain : Gain  Gain=Kp_ROLL_ANGLE
  y : Outport  InitialOutput=0
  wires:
  Gain/1 -> y/1
  x/1 -> Gain/1

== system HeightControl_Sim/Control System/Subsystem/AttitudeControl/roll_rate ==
  x : Inport
  reset_i : Inport  Port=2
  Derivative Gain : Gain  DisableCoverage=on  Gain=Kd_ROLL_AngleRate  ParamMin=-100  ParamMax=100  OutMin=-100  OutMax=100
  Discrete Derivative : simulink/Discrete/Discrete Derivative  gainval=1.0  ICPrevScaledInput=0.0  OutMin=[]  OutMax=[]  OutDataType=fixdt(1, 16)  OutScaling=2^-10  DoSatur=off
  Discrete-Time Integrator : DiscreteIntegrator  ExternalReset=level  InitialConditionSetting=State (most efficient)  SampleTime=-1  LimitOutput=on  UpperSaturationLimit=Saturation_I_RP_Max  LowerSaturationLimit=Saturation_I_RP_Min  ICPrevOutput=DiscIntNeverNeededParam  ICPrevScaledInput=DiscIntNeverNeededParam
  Gain : Gain  Gain=Kp_ROLL_AngleRate
  Integral Gain : Gain  DisableCoverage=on  Gain=Ki_ROLL_AngleRate
  Sum : Sum  Inputs=+++
  y : Outport  InitialOutput=0
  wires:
  x/1 -> Gain/1, Integral Gain/1, Derivative Gain/1
  Integral Gain/1 -> Discrete-Time Integrator/1
  Derivative Gain/1 -> Discrete Derivative/1
  Gain/1 -> Sum/1
  Sum/1 -> y/1
  Discrete Derivative/1 -> Sum/3
  Discrete-Time Integrator/1 -> Sum/2
  reset_i/1 -> Discrete-Time Integrator/2

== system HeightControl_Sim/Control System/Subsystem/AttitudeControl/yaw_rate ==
  x : Inport
  reset_i : Inport  Port=2
  Derivative Gain : Gain  DisableCoverage=on  Gain=Kd_YAW_AngleRate  ParamMin=-100  ParamMax=100  OutMin=-100  OutMax=100
  Discrete Derivative : simulink/Discrete/Discrete Derivative  gainval=1.0  ICPrevScaledInput=0.0  OutMin=[]  OutMax=[]  OutDataType=fixdt(1, 16)  OutScaling=2^-10  DoSatur=off
  Discrete-Time Integrator : DiscreteIntegrator  ExternalReset=level  InitialConditionSetting=State (most efficient)  SampleTime=-1  LimitOutput=on  UpperSaturationLimit=Saturation_I_Y_Max  LowerSaturationLimit=Saturation_I_Y_Min  ICPrevOutput=DiscIntNeverNeededParam  ICPrevScaledInput=DiscIntNeverNeededParam
  Gain : Gain  Gain=Kp_YAW_AngleRate
  Integral Gain : Gain  DisableCoverage=on  Gain=Ki_YAW_AngleRate
  Sum : Sum  Inputs=+++
  y : Outport  InitialOutput=0
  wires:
  x/1 -> Gain/1, Integral Gain/1, Derivative Gain/1
  Integral Gain/1 -> Discrete-Time Integrator/1
  Derivative Gain/1 -> Discrete Derivative/1
  Gain/1 -> Sum/1
  Sum/1 -> y/1
  Discrete Derivative/1 -> Sum/3
  Discrete-Time Integrator/1 -> Sum/2
  reset_i/1 -> Discrete-Time Integrator/2

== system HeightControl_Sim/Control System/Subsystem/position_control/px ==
  ex : Inport
  Gain1 : Gain  Gain=Kpxp
  Saturation3 : Saturate  UpperLimit=MAX_CONTROL_VELOCITY_XY  LowerLimit=-MAX_CONTROL_VELOCITY_XY
  vxd : Outport
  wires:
  ex/1 -> Gain1/1
  Saturation3/1 -> vxd/1
  Gain1/1 -> Saturation3/1

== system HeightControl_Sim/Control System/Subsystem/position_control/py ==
  ey : Inport
  Gain1 : Gain  Gain=Kpyp
  Saturation3 : Saturate  UpperLimit=MAX_CONTROL_VELOCITY_XY  LowerLimit=-MAX_CONTROL_VELOCITY_XY
  vyd : Outport
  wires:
  Gain1/1 -> Saturation3/1
  Saturation3/1 -> vyd/1
  ey/1 -> Gain1/1

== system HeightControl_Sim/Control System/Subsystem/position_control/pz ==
  ez : Inport
  Gain1 : Gain  Gain=Kpzp
  Saturation3 : Saturate  UpperLimit=MAX_CONTROL_VELOCITY_Z  LowerLimit=-MAX_CONTROL_VELOCITY_Z
  vzd : Outport
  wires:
  ez/1 -> Gain1/1
  Saturation3/1 -> vzd/1
  Gain1/1 -> Saturation3/1

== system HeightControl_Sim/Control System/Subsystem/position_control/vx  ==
  x : Inport
  reset_i : Inport  Port=2
  Derivative Gain : Gain  DisableCoverage=on  Gain=Kvxd
  Discrete Derivative : simulink/Discrete/Discrete Derivative  gainval=1.0  ICPrevScaledInput=0.0  OutMin=[]  OutMax=[]  OutDataType=fixdt(1, 16)  OutScaling=2^-10  DoSatur=off
  Discrete-Time Integrator : DiscreteIntegrator  ExternalReset=level  InitialConditionSetting=State (most efficient)  SampleTime=-1  LimitOutput=on  UpperSaturationLimit=Saturation_I_ah  LowerSaturationLimit=-Saturation_I_ah  ICPrevOutput=DiscIntNeverNeededParam  ICPrevScaledInput=DiscIntNeverNeededParam
  Gain : Gain  Gain=Kvxp
  Integral Gain : Gain  DisableCoverage=on  Gain=Kvxi
  Sum : Sum  Inputs=+++
  y : Outport  InitialOutput=0
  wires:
  x/1 -> Gain/1, Integral Gain/1, Derivative Gain/1
  Integral Gain/1 -> Discrete-Time Integrator/1
  Derivative Gain/1 -> Discrete Derivative/1
  Gain/1 -> Sum/1
  Sum/1 -> y/1
  Discrete Derivative/1 -> Sum/3
  Discrete-Time Integrator/1 -> Sum/2
  reset_i/1 -> Discrete-Time Integrator/2

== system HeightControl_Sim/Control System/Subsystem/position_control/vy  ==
  x : Inport
  reset_i : Inport  Port=2
  Derivative Gain : Gain  DisableCoverage=on  Gain=Kvyd
  Discrete Derivative : simulink/Discrete/Discrete Derivative  gainval=1.0  ICPrevScaledInput=0.0  OutMin=[]  OutMax=[]  OutDataType=fixdt(1, 16)  OutScaling=2^-10  DoSatur=off
  Discrete-Time Integrator : DiscreteIntegrator  ExternalReset=level  InitialConditionSetting=State (most efficient)  SampleTime=-1  LimitOutput=on  UpperSaturationLimit=Saturation_I_ah  LowerSaturationLimit=-Saturation_I_ah  ICPrevOutput=DiscIntNeverNeededParam  ICPrevScaledInput=DiscIntNeverNeededParam
  Gain : Gain  Gain=Kvyp
  Integral Gain : Gain  DisableCoverage=on  Gain=Kvyi
  Sum : Sum  Inputs=+++
  y : Outport  InitialOutput=0
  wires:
  x/1 -> Gain/1, Integral Gain/1, Derivative Gain/1
  Integral Gain/1 -> Discrete-Time Integrator/1
  Derivative Gain/1 -> Discrete Derivative/1
  Gain/1 -> Sum/1
  Sum/1 -> y/1
  Discrete Derivative/1 -> Sum/3
  Discrete-Time Integrator/1 -> Sum/2
  reset_i/1 -> Discrete-Time Integrator/2

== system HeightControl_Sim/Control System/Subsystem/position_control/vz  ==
  x : Inport
  reset_i : Inport  Port=2
  Derivative Gain : Gain  DisableCoverage=on  Gain=Kvzd
  Discrete Derivative : simulink/Discrete/Discrete Derivative  gainval=1.0  ICPrevScaledInput=0.0  OutMin=[]  OutMax=[]  OutDataType=fixdt(1, 16)  OutScaling=2^-10  DoSatur=off
  Discrete-Time Integrator : DiscreteIntegrator  ExternalReset=level  InitialConditionSetting=State (most efficient)  SampleTime=-1  LimitOutput=on  UpperSaturationLimit=Saturation_I_az  LowerSaturationLimit=-Saturation_I_az  ICPrevOutput=DiscIntNeverNeededParam  ICPrevScaledInput=DiscIntNeverNeededParam
  Gain : Gain  Gain=Kvzp
  Integral Gain : Gain  DisableCoverage=on  Gain=Kvzi
  Sum : Sum  Inputs=+++
  y : Outport  InitialOutput=0
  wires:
  Discrete-Time Integrator/1 -> Sum/2
  Discrete Derivative/1 -> Sum/3
  Sum/1 -> y/1
  Gain/1 -> Sum/1
  Derivative Gain/1 -> Discrete Derivative/1
  Integral Gain/1 -> Discrete-Time Integrator/1
  x/1 -> Derivative Gain/1, Integral Gain/1, Gain/1
  reset_i/1 -> Discrete-Time Integrator/2

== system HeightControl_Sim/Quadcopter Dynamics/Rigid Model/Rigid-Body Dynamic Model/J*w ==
  p q r : Inport
  J : Inport  Port=2
  J*w : Product  Multiplication=Matrix(*)
  "J*w " : Outport
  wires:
  J*w/1 -> "J*w "/1
  J/1 -> J*w/1
  p q r/1 -> J*w/2

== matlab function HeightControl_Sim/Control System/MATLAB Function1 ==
function reset_i= fcn(ch3)
%Function description:
%  reset Integral when throttle < 1250
if ch3<1250
    reset_i=[1 1 1 1];
else
    reset_i=[0 0 0 0];
end

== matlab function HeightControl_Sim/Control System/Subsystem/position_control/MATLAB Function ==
function [phi, theta] = fcn(eax, eay, psi)
%Function description:
%  Convert the desired horizontal acceleration to the desired Euler angle.
%Input:
%  eax, eay: desired horizontal acceleration
%  psi: yaw
%Output:
%  phi, theta: desired roll and pitch
g = 9.8;
phi = (-sin(psi)*eax + cos(psi)*eay)/g;
theta = (-cos(psi)*eax - sin(psi)*eay)/g;

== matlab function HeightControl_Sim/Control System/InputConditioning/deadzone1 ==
function y = fcn(u)
%Function description:
%  Control the range of the remote control input from RCMin to RCMax, and
%  set a dead zone with a dead zone size of ±deadZone. The output y is
%  normalized to 0~1.You can get the RC calibration parameters in QGC.
RCMin = 1100;
RCMax = 1900;
RCMid = (RCMin + RCMax)/2;
deadZoneRate = 0.05;
deadZone = deadZoneRate*(RCMax - RCMin);
k = 1/(RCMax - RCMid - deadZone);
% saturation
if(u < RCMin)
    u = RCMin;
elseif(u > RCMax)
    u = RCMax;
end
% dead zone and normalize
 if(u > RCMid + deadZone)
    y = (u-RCMid - deadZone)*k;
 elseif(u < RCMid - deadZone)
     y = (u - RCMid + deadZone)*k;
 else
     y = 0;
 end

 end

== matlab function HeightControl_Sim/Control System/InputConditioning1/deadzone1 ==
function y = fcn(u)
%Function description:
%  Control the range of the remote control input from RCMin to RCMax, and
%  set a dead zone with a dead zone size of ±deadZone. The output y is
%  normalized to 0~1.You can get the RC calibration parameters in QGC.
RCMin = 1100;
RCMax = 1900;
RCMid = (RCMin + RCMax)/2;
deadZoneRate = 0.05;
deadZone = deadZoneRate*(RCMax - RCMin);
k = 1/(RCMax - RCMid - deadZone);
% saturation
if(u < RCMin)
    u = RCMin;
elseif(u > RCMax)
    u = RCMax;
end
% dead zone and normalize
 if(u > RCMid + deadZone)
    y = (u-RCMid - deadZone)*k;
 elseif(u < RCMid - deadZone)
     y = (u - RCMid + deadZone)*k;
 else
     y = 0;
 end

 end

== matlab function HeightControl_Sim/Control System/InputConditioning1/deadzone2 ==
function y = fcn(u)
%Function description:
%  Control the range of the remote control input from RCMin to RCMax, and
%  set a dead zone with a dead zone size of ±deadZone. The output y is
%  normalized to 0~1.You can get the RC calibration parameters in QGC.
RCMin = 1100;
RCMax = 1900;
RCMid = (RCMin + RCMax)/2;
deadZoneRate = 0.05;
deadZone = deadZoneRate*(RCMax - RCMin);
k = 1/(RCMax - RCMid - deadZone);
% saturation
if(u < RCMin)
    u = RCMin;
elseif(u > RCMax)
    u = RCMax;
end
% dead zone and normalize
 if(u > RCMid + deadZone)
    y = (u-RCMid - deadZone)*k;
 elseif(u < RCMid - deadZone)
     y = (u - RCMid + deadZone)*k;
 else
     y = 0;
 end

 end

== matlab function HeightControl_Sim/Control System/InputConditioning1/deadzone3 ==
function y = fcn(u)
%Function description:
%  Control the range of the remote control input from RCMin to RCMax, and
%  set a dead zone with a dead zone size of ±deadZone. The output y is
%  normalized to 0~1.You can get the RC calibration parameters in QGC.
RCMin = 1100;
RCMax = 1900;
RCMid = (RCMin + RCMax)/2;
deadZoneRate = 0.05;
deadZone = deadZoneRate*(RCMax - RCMin);
k = 1/(RCMax - RCMid - deadZone);
% saturation
if(u < RCMin)
    u = RCMin;
elseif(u > RCMax)
    u = RCMax;
end
% dead zone and normalize
 if(u > RCMid + deadZone)
    y = (u-RCMid - deadZone)*k;
 elseif(u < RCMid - deadZone)
     y = (u - RCMid + deadZone)*k;
 else
     y = 0;
 end

 end

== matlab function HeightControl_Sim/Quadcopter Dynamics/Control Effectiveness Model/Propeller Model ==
function [Fb, Fd, Mb, Md, Ga] = fcn(w, R, Cm, Ct, Vb, Cd,wb, Cdm, Jrp)
 %Function description:
 %  Obtain the force and torque acting on the body. The airframe of the
 %  quadrotor is as follows:
 %3↓   1↑
 %  \ /
 %  / \
 %2↑   4↓
 %↑ stands for counterclockwise and ↓stands for clockwise.
 %Input：
 %  w: motor speed，unit：rad/s
 %  R: body radius(m)
 %  Cm: torque coefficient
 %  Ct: thrust coefficient
 %  Vb: aircraft speed in the body coordinate system
 %  Cd: damping coefficient
 %  wb: angular velocity in the body coordinate system
 %  Cdm: damping moment coefficient vector
 %  Jrp:  moment of inertia of motor rotor + propeller
 %Output:
 %  Fb: thrust under the body coordinate system
 %  Fd: aerodynamic force under the body coordinate system
 %  Mb: torque under the body coordinate system
 %  Md: aerodynamic moment
 %  Ga: gyro moment
 M_rctcm = [-sin(pi/4)*R*Ct, sin(pi/4)*R*Ct, sin(pi/4)*R*Ct, -sin(pi/4)*R*Ct;
            sin(pi/4)*R*Ct, -sin(pi/4)*R*Ct, sin(pi/4)*R*Ct, -sin(pi/4)*R*Ct;
            Cm, Cm, -Cm, -Cm];
 Mb = M_rctcm*(w.^2);  % torque
 
 Fb = [0; 0; -sum(Ct*(w.^2))];  % thrust
 Fd = -Cd*Vb.*abs(Vb)*0.5;  % aerodynamic force
 Md = -Cdm.*wb.*abs(wb);  % aerodynamic moment
 % gyro moment
 Ga = zeros(3,1);
 Ga(1) = Jrp*wb(2)*( w(1) + w(2) - w(3) - w(4));
 Ga(2) = Jrp*wb(1)*(-w(1) - w(2) + w(3) + w(4));
end

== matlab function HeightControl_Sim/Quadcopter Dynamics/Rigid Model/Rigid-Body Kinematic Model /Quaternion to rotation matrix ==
function Reb = fcn(q)
%Function description;
%  The rotation matrix of the Aircraft-Body Coordinate Frame (ABCF) to the
%  Earth-Fixed Coordinate Frame (EFCF) is obtained from the quaternions
Reb = [q(1)*q(1) + q(2)*q(2) - q(3)*q(3) - q(4)*q(4), 2*(q(2)*q(3) - q(1)*q(4)), 2*(q(2)*q(4) + q(1)*q(3))
           2*(q(2)*q(3) + q(1)*q(4)), q(1)*q(1) - q(2)*q(2) + q(3)*q(3) - q(4)*q(4), 2*(q(3)*q(4) - q(1)*q(2))
           2*(q(2)*q(4) - q(1)*q(3)), 2*(q(3)*q(4) + q(1)*q(2)), q(1)*q(1) - q(2)*q(2) - q(3)*q(3) + q(4)*q(4)];

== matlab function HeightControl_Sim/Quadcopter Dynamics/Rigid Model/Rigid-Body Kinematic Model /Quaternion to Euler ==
function y = fcn(q)
 %Function description:
%  Quaternions to Euler
phi = atan2(2*(q(1)*q(2) + q(3)*q(4)), (1 - 2*(q(2)*q(2) + q(3)*q(3))));
theta = asin(2*(q(1)*q(3) - q(2)*q(4)));
psi = atan2(2*(q(1)*q(4) + q(2)*q(3)), (1 - 2*(q(3)*q(3) + q(4)*q(4))));
y = [phi theta psi];

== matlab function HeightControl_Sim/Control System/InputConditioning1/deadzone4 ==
function y = fcn(u)
%Function description:
%  Control the range of the remote control input from RCMin to RCMax, and
%  set a dead zone with a dead zone size of ±deadZone. The output y is
%  normalized to 0~1.You can get the RC calibration parameters in QGC.
RCMin = 1100;
RCMax = 1900;
RCMid = (RCMin + RCMax)/2;
deadZoneRate = 0.05;
deadZone = deadZoneRate*(RCMax - RCMin);
k = 1/(RCMax - RCMid - deadZone);
% saturation
if(u < RCMin)
    u = RCMin;
elseif(u > RCMax)
    u = RCMax;
end
% dead zone and normalize
 if(u > RCMid + deadZone)
    y = (u-RCMid - deadZone)*k;
 elseif(u < RCMid - deadZone)
     y = (u - RCMid + deadZone)*k;
 else
     y = 0;
 end

 end

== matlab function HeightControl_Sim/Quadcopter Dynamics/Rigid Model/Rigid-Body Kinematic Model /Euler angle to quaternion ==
function q = fcn(EulerAngle)
%Function description:
%  Get quaternions from Euler angle
q0 =  cos(EulerAngle(1)/2)*cos(EulerAngle(2)/2)*cos(EulerAngle(3)/2) + sin(EulerAngle(1)/2)*sin((EulerAngle(2)/2))*sin((EulerAngle(3)/2));
q1 = sin(EulerAngle(1)/2)*cos(EulerAngle(2)/2)*cos(EulerAngle(3)/2) - cos(EulerAngle(1)/2)*sin((EulerAngle(2)/2))*sin((EulerAngle(3)/2));
q2 = cos(EulerAngle(1)/2)*sin(EulerAngle(2)/2)*cos(EulerAngle(3)/2) + sin(EulerAngle(1)/2)*cos((EulerAngle(2)/2))*sin((EulerAngle(3)/2));
q3 = cos(EulerAngle(1)/2)*cos(EulerAngle(2)/2)*sin(EulerAngle(3)/2) - sin(EulerAngle(1)/2)*sin((EulerAngle(2)/2))*cos((EulerAngle(3)/2));
q = [q0 q1 q2 q3]';
